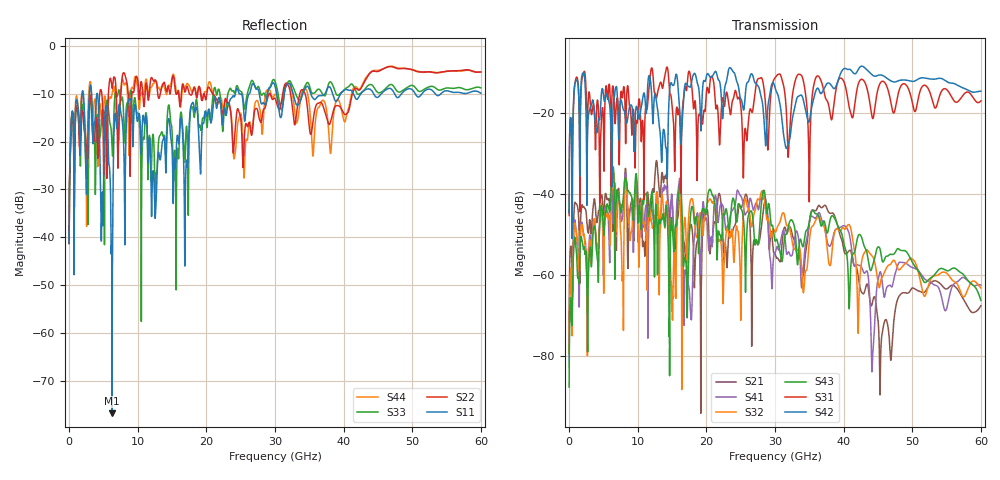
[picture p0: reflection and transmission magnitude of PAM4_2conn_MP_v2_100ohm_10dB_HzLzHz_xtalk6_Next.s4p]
! Info: Touchstone file created by Circ.  Input file=FAB50GbE_2conn_Midplane_Examax_Topo2_v2_100ohm_10dB_HzLzHz.circ
# Hz S RI R 50
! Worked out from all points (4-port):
!   6000 points, 10 MHz to 60 GHz, reference 50 ohm
!   strongest paths, dB at 10 MHz, 15.01 GHz, 30.01 GHz, 45.01 GHz, 60 GHz:
!     S42: -44.6, -12.9, -13.6, -10.6, -14.5
!     S31: -45.2, -18.1, -11.2, -14.0, -16.9
!     S43: -87.6, -47.6, -51.5, -53.0, -66.2
!     S32: -79.1, -68.5, -49.2, -61.6, -63.1
!     S41: -82.7, -40.6, -54.4, -61.1, -62.4
!     S21: -77.6, -41.9, -54.7, -71.0, -67.5
!   lowest |S11| = -76.7 dB at 6.28 GHz (marker M1), VSWR 1.00, Z = 50 - j0.00605 ohm
!   |S11| at or under -10 dB: start of sweep to 1.888 GHz; 4.127 GHz to 24.22 GHz (20.09 GHz wide, 142 % of centre); 35.21 GHz to 37.29 GHz (2.083 GHz wide, 5.75 % of centre)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
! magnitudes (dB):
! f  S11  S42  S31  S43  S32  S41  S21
! 10 MHz  -41.2  -44.6  -45.2  -87.6  -79.1  -82.7  -77.6
! 3.11 GHz  -8.2  -18.4  -17.7  -53.1  -52.0  -50.7  -47.7
! 6.28 GHz  -76.7  -28.5  -14.6  -35.7  -38.0  -38.1  -41.1
! 8.8 GHz  -11.1  -18.5  -18.1  -39.6  -48.7  -45.4  -44.0
! 40.17 GHz  -9.2  -8.9  -12.8  -52.9  -48.6  -47.7  -54.5
! 44.24 GHz  -9.7  -10.6  -21.3  -57.5  -55.4  -79.5  -66.3
! 60 GHz  -9.9  -14.5  -16.9  -66.2  -63.1  -62.4  -67.5
